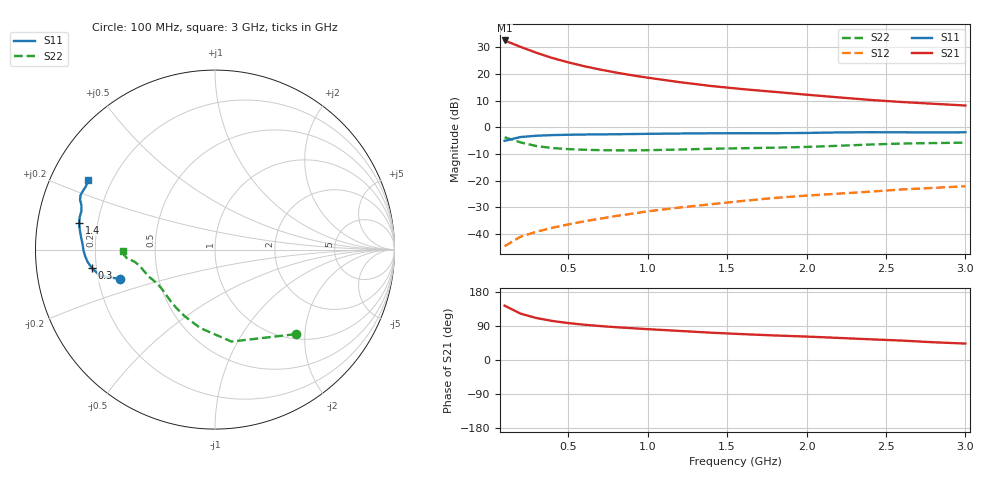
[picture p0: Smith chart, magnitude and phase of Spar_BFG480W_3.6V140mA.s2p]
! Filename: 3_6140BFG480.001
! Title: BFG480W
! Bias: Vce=3.6V; Ic=140mA
! Company: NXP Semiconductors NL
! User: Quality&Reliability T&D
! Measure time: 10 Nov 1999 / 12:01:48
#  MHz  S  MA  R 50
! Freq  S11  S21  S12  S22  :
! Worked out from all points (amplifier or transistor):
!   20 points, 100 MHz to 3 GHz, reference 50 ohm
!   highest |S21| = 32.6 dB at 100 MHz (marker M1)
!   |S21| within 3 dB of that: start of sweep to 226.9 MHz
!   unconditionally stable (mu >= 1): 485.7 MHz to end of sweep
!   at 400 MHz: K = 0.95, MSG = 31.9 dB, |S12| = -37.8 dB
!   at 1.2 GHz: K = 1.12, MAG = 21.4 dB, |S12| = -30.2 dB
!   at 3 GHz: K = 1.08, MAG = 13.4 dB, |S12| = -22.1 dB
!   S11 on the Smith chart (normalised r, x): 100 MHz: 0.29, -0.14; 300 MHz: 0.18, -0.07; 1.4 GHz: 0.13, +0.10; 3 GHz: 0.11, +0.25
100  0.5565 -162.9  42.8 143.4  0.005845 67.6  0.6505 -46.4
200  0.6563 -167.2  32.46 122.5  0.008798 60.6  0.5205 -79.8
300  0.6939 -171.5  25.15 110.8  0.0109 61.1  0.4448 -100.6
400  0.7138 -174.6  20.06 103.0  0.01295 63.7  0.4079 -114.4
500  0.7245 -177.2  16.62 97.5  0.01496 66.3  0.3892 -124.0
600  0.7317 -179.3  14.06 93.1  0.0171 68.3  0.3786 -131.0
700  0.7358 178.8  12.19 89.6  0.01921 70.2  0.3722 -136.2
800  0.7407 177.0  10.7 86.6  0.02154 71.8  0.369 -140.6
900  0.7472 175.3  9.505 83.9  0.02378 73.5  0.3686 -144.4
1000  0.7534 173.7  8.554 81.4  0.02637 74.3  0.3712 -147.7
1200  0.7644 170.9  7.058 76.7  0.03107 75.7  0.3824 -153.1
1400  0.7718 168.7  5.97 72.1  0.03588 76.4  0.3954 -157.0
1600  0.7754 166.4  5.207 68.2  0.04136 76.8  0.4043 -160.1
1800  0.7743 163.9  4.629 64.8  0.04718 77.1  0.4142 -163.5
2000  0.7831 161.8  4.097 61.8  0.05206 77.6  0.4281 -167.6
2200  0.8013 159.8  3.652 58.3  0.05669 77.4  0.4494 -171.0
2400  0.8083 158.0  3.269 54.6  0.06174 76.7  0.4746 -173.2
2600  0.8056 156.2  2.985 51.2  0.06799 75.9  0.4949 -174.6
2800  0.8008 153.9  2.766 46.8  0.07278 74.3  0.5057 -176.4
3000  0.8059 151.2  2.568 43.4  0.07825 73.5  0.5146 -179.2
